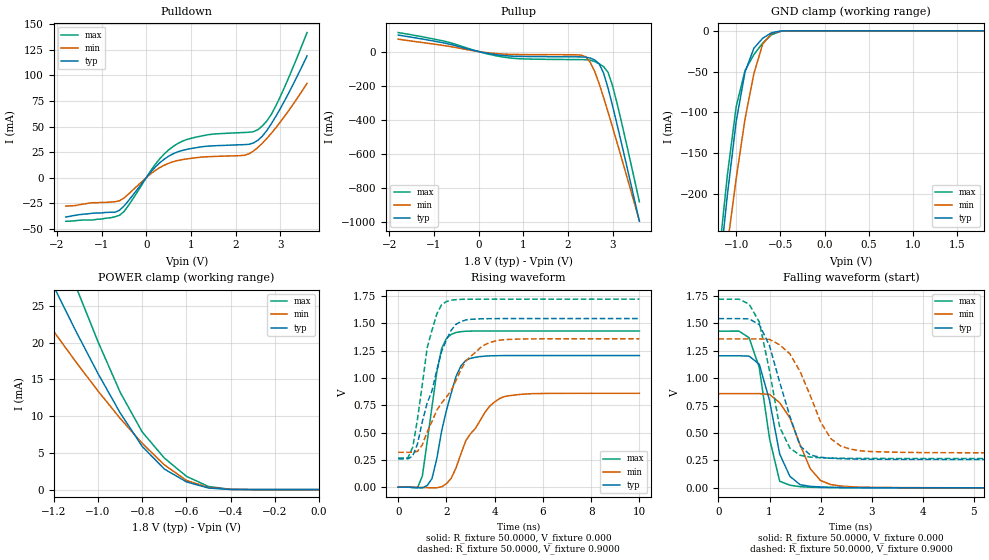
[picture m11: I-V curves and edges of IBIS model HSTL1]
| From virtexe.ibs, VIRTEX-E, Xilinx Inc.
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|   Model HSTL1
[Model]   HSTL1
Model_type   I/O
Polarity   Non-Inverting
Enable   Active-Low
Vinl =  0.8000V
Vinh =  1.0000V
Vmeas =   0.9000V
Cref =  20.0000pF
Rref =  50.0000
Vref =   0.9000V
C_comp   6.0000pF   5.0000pF   7.0000pF
[Temperature Range]   25.0000   100.0000   0.000
[Voltage Range]   1.8000V   1.7000V   1.9000V
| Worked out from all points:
|   slope of the pulldown table from 0 to 0.27 V, typ, clamps not added: 20.5 ohm
|   slope of the pullup table from 0 to 0.27 V, typ, clamps not added: 20.1 ohm
|   GND clamp passes 1 mA (typ) near -0.54 V on its own axis
|   POWER clamp passes 1 mA (typ) near -0.59 V on its own axis
|   rising waveform, R_fixture 50.0000, V_fixture 0.000: 20-80 % time 753ps typ, 1.22ns min, 566ps max; typ from 0 V to 1.21 V
|   rising waveform, R_fixture 50.0000, V_fixture 0.9000: 20-80 % time 965ps typ, 1.55ns min, 644ps max; typ from 0.259 V to 1.54 V
|   falling waveform, R_fixture 50.0000, V_fixture 0.000: 20-80 % time 367ps typ, 476ps min, 319ps max; typ from 1.21 V to 0 V
|   falling waveform, R_fixture 50.0000, V_fixture 0.9000: 20-80 % time 495ps typ, 610ps min, 361ps max; typ from 1.54 V to 0.259 V
[Pulldown]
| voltage   I(typ)   I(min)   I(max)
-1.8V     -38.5mA    -27.8mA    -42.7mA
-600mV    -31.92mA   -22.63mA   -36.84mA
-400mV    -22.62mA   -16.13mA   -27.31mA
200mV     10.29mA    6.956mA    12.96mA
500mV     20.93mA    14.03mA    27.05mA
800mV     26.54mA    17.58mA    35.49mA
1.4V      30.87mA    20.52mA    42.1mA
2.2V      32.29mA    21.92mA    44.18mA
2.5V      36.57mA    29.54mA    46.93mA
2.7V      46.1mA     38.33mA    55.43mA
2.9V      59.8mA     48.7mA     70.05mA
3.6V      119.1mA    92.2mA     141.9mA
[Pullup]
| voltage   I(typ)   I(min)   I(max)
-1.8V     97.04mA    72.78mA    111.7mA
-800mV    51.88mA    36.3mA     62.98mA
600mV     -24.24mA   -15.32mA   -34.04mA
2.3V      -31.3mA    -20.95mA   -47.36mA
2.4V      -32.73mA   -30.87mA   -47.8mA
2.6V      -49.01mA   -116.6mA   -58.63mA
2.7V      -71.91mA   -188.9mA   -71.8mA
2.8V      -127.2mA   -270.6mA   -88.68mA
2.9V      -216mA     -356.6mA   -122.6mA
3V        -319mA     -444.8mA   -201.1mA
3.2V      -539.1mA   -625.1mA   -414.5mA
3.6V      -997.5mA   -993.6mA   -882.6mA
[GND_clamp]
| voltage   I(typ)   I(min)   I(max)
-1.8V     -984.2mA   -893.8mA   -981.3mA
-1.2V     -305.4mA   -349.4mA   -281.7mA
-1.1V     -201.6mA   -263.3mA   -177.2mA
-1V       -111.1mA   -181.2mA   -92.91mA
-900mV    -50.62mA   -108.2mA   -48.68mA
-800mV    -21.39mA   -52.51mA   -29.19mA
-700mV    -9.057mA   -16.26mA   -15mA
-600mV    -2.332mA   -3.044mA   -4.887mA
-500mV    -280.5uA   -493uA     -684.1uA
-400mV    -21.31uA   -72.94uA   -46.93uA
1.8V      9.75nA     24.68nA    9.371nA
[POWER_clamp]
| voltage   I(typ)   I(min)   I(max)
-1.8V     67.36mA    47.92mA    87.19mA
-1.3V     33.96mA    25.81mA    43.76mA
-1.2V     27.64mA    21.52mA    35.56mA
-1.1V     21.56mA    17.38mA    27.65mA
-1V       15.79mA    13.42mA    20.13mA
-900mV    10.45mA    9.702mA    13.26mA
-800mV    5.872mA    6.297mA    7.84mA
-700mV    2.804mA    3.371mA    4.298mA
-600mV    1.052mA    1.252mA    1.806mA
-500mV    210uA      278.7uA    420.1uA
-400mV    17.08uA    35.57uA    36.55uA
0V        9.75nA     16.07nA    10.24nA
[Ramp]
| variable   typ   min   max
dV/dt_r   0.7230/0.7418n   0.5158/1.2132n   0.8580/0.4812n
dV/dt_f   0.7095/0.6353n   0.5303/0.9472n   0.8297/0.4699n
R_load = 50.0000
[Rising Waveform]
R_fixture = 50.0000
V_fixture = 0.000
| time   V(typ)   V(min)   V(max)
0s        0V         0V         1.326uV
800ps     -5.897mV   -1.125mV   -4.456mV
1ns       -6.477mV   -3.129mV   100.5mV
1.4ns     78.01mV    -6.314mV   735.7mV
1.6ns     260.2mV    -5.42mV    1.053V
1.8ns     514mV      3.223mV    1.269V
2.2ns     863.2mV    81.35mV    1.399V
2.8ns     1.16V      423.4mV    1.428V
4.2ns     1.204V     811.2mV    1.43V
10ns      1.205V     859.6mV    1.43V
[Rising Waveform]
R_fixture = 50.0000
V_fixture = 0.9000
V_fixture_min = 0.8300
V_fixture_max = 1.1000
| time   V(typ)   V(min)   V(max)
0s        259mV      318.9mV    267.1mV
400ps     259.8mV    319mV      268.7mV
600ps     284.4mV    319.3mV    363.7mV
1ns       600.5mV    388.6mV    940.3mV
1.2ns     769.1mV    504.1mV    1.275V
1.8ns     1.243V     771mV      1.671V
2.4ns     1.492V     979.5mV    1.718V
2.8ns     1.531V     1.152V     1.721V
3.8ns     1.543V     1.325V     1.722V
10ns      1.544V     1.359V     1.722V
[Falling Waveform]
R_fixture = 50.0000
V_fixture = 0.000
| time   V(typ)   V(min)   V(max)
0s        1.205V     859.6mV    1.43V
400ps     1.205V     859.6mV    1.431V
600ps     1.202V     859.6mV    1.37V
800ps     1.128V     859.8mV    1.096V
1ns       798.4mV    852.7mV    451.2mV
1.2ns     308.2mV    777.1mV    60.04mV
1.4ns     105.3mV    637.4mV    24.72mV
1.8ns     13.66mV    174.3mV    5.816mV
2.2ns     4.997mV    30.1mV     2.413mV
10ns      154.3uV    281.7uV    126.5uV
[Falling Waveform]
R_fixture = 50.0000
V_fixture = 0.9000
V_fixture_min = 0.8300
V_fixture_max = 1.1000
| time   V(typ)   V(min)   V(max)
0s        1.544V     1.359V     1.722V
600ps     1.542V     1.359V     1.677V
800ps     1.49V      1.359V     1.513V
1ns       1.297V     1.355V     1.068V
1.2ns     962.6mV    1.305V     553.6mV
1.4ns     652.5mV    1.222V     363.1mV
1.6ns     382.2mV    1.062V     297.5mV
2.2ns     270.4mV    449.2mV    271.6mV
2.6ns     263.7mV    352.3mV    269.2mV
10ns      259.2mV    319.3mV    267.3mV
